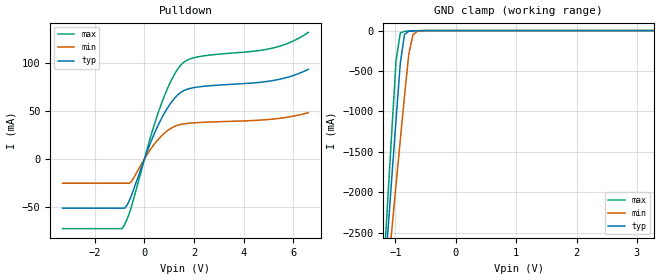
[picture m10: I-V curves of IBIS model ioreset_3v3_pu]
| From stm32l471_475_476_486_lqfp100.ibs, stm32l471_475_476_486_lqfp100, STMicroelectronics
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|   Model ioreset_3v3_pu
[Model]  ioreset_3v3_pu
Model_type I/O_open_drain
Polarity   Inverting
Enable   Active-High
Vinl =   0.990000V
Vinh =   2.310000V
Vmeas =  1.650000V
Cref =   100.000000nF
Rref =   1.000000k
Vref =   3.300000V
C_comp   0.541680pF   0.532160pF   0.622160pF
[Temperature Range]   25.000000   0.125000k   -40.000000
[Pullup Reference]   3.300000V   2.700000V   3.600000V
[Pulldown Reference]   0.0V   0.0V   0.0V
[POWER Clamp Reference]   3.300000V   2.700000V   3.600000V
[GND Clamp Reference]   0.0V   0.0V   0.0V
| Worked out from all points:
|   slope of the pulldown table from 0 to 0.495 V, typ, clamps not added: 15.4 ohm
|   GND clamp passes 1 mA (typ) near -0.59 V on its own axis
[Pulldown]
|Voltage   I(typ)   I(min)   I(max)
-3.3V     -51.63mA   -25.53mA   -73.04mA
-900mV    -51.63mA   -25.53mA   -73.04mA
-700mV    -48.45mA   -25.53mA   -63.02mA
-500mV    -36.51mA   -22.8mA    -47.71mA
200mV     14.03mA    8.316mA    18.9mA
700mV     42.99mA    24.4mA     58.9mA
1.2V      63.06mA    33.8mA     88.14mA
1.6V      71.64mA    36.67mA    101.4mA
2.3V      75.63mA    38.12mA    107.4mA
5.2V      82.02mA    41.68mA    116.1mA
5.9V      86.41mA    44.22mA    122.2mA
6.6V      93.66mA    48.27mA    132.3mA
[GND_clamp]
|Voltage   I(typ)   I(min)   I(max)
-3.3V     -9.812A    -9.988A    -9.329A
-1.2V     -3.251A    -3.583A    -3.017A
-1.13V    -2.528A    -3.02A     -2.122A
-1.06V    -1.808A    -2.459A    -1.234A
-990mV    -1.097A    -1.901A    -369.4mA
-920mV    -404.3mA   -1.349A    -29.79mA
-850mV    -46.63mA   -808.1mA   -9.867mA
-780mV    -8.596mA   -293.7mA   -6.34mA
-710mV    -3.483mA   -50.92mA   -3.779mA
-640mV    -1.689mA   -10.39mA   -1.818mA
-430mV    -117.5uA   -209uA     -95.53uA
3.28V     0A         0A         0A
[POWER_clamp]
|Voltage   I(typ)   I(min)   I(max)
-3.28V    0A         0A         0A
0V        0A         0A         0A
[Ramp]
| variable   typ   min   max
dV/dt_r  1.97933/0.10397u   1.61897/0.10190u   2.15945/0.10455u
dV/dt_f  1.97933/5.68063n   1.61903/9.19249n   2.15945/4.39416n
R_load = 40.000000k
